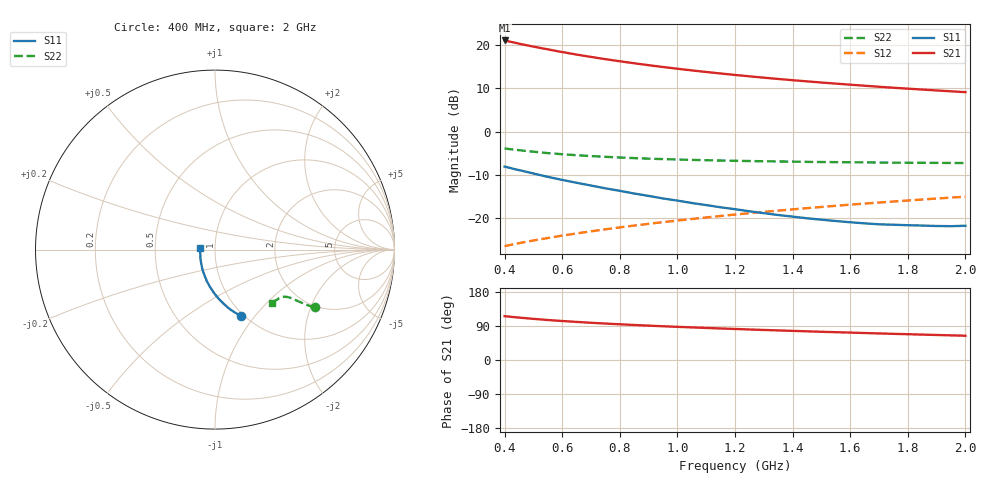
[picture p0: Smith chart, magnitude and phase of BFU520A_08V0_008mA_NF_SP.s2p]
! Filename:  P:\Prog\Test\Noise\ATS_data\Testdata_Net\06 Compressed Noise after Statistics\BFU520A_APG2013_30_A05_08p0V_008mA_NF_CM01_D.sf
! Date/Time: Wed 24/Apr/2013 20:06:19
! BFU520A_APG2013_30_A05_08p0V_1to20mA_NF_CM01_Bias5_R.sf
! Noise Parameter Data File
! BFU520A_APG2013_30_A05_08p0V_1to20mA_NF_CM01
! Date/time: Thu Apr 11 09:33:54 2013
! VAR V_out= 8.000000
! VAR I_out= 8.005000
! VAR V_in= 0.828700
! VAR I_in= 0.085505
! Device data file deembeded for feedlines and parallel
! Original file: \06 Compressed Noise after Statistics\BFU520A_APG2013_30_A05_08p0V_008mA_NF_CM01_R.sf
! Feed-files: PR017V01_150413_Feed1.s2p, PR017V01_150413_Feed2.s2p
! Parallel-file: PR017V01_150413_Par.s2p
# MHz S MA R 50
!  Freq-MHz  S11-mag  S11-arg  S21-mag  S21-arg  S12-mag  S12-arg  S22-mag  S22-arg
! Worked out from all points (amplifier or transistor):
!   37 points, 400 MHz to 2 GHz, reference 50 ohm
!   highest |S21| = 21.1 dB at 400 MHz (marker M1)
!   |S21| within 3 dB of that: start of sweep to 627.7 MHz
!   unconditionally stable (mu >= 1): 1.423 GHz to end of sweep
!   at 500 MHz: K = 0.76, MSG = 22.4 dB, |S12| = -25.1 dB
!   at 1.1 GHz: K = 0.97, MSG = 16.8 dB, |S12| = -19.8 dB
!   at 2 GHz: K = 1.01, MAG = 11.6 dB, |S12| = -15.0 dB
!   lowest NFmin = 0.76 dB at 420 MHz
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400  0.3961 -68.7  11.34 115.7  0.0478 67.2  0.6417 -30.1
420  0.3819 -70.6  10.95 114.1  0.04942 67.1  0.6294 -30.4
440  0.3676 -72.5  10.6 112.6  0.051 67.1  0.6184 -30.6
460  0.3549 -74.1  10.25 111.2  0.05255 67.2  0.6082 -30.9
480  0.3424 -75.9  9.927 109.9  0.05409 67.1  0.5977 -31.1
500  0.3301 -77.5  9.621 108.6  0.05564 67.2  0.589 -31.2
550  0.3016 -81.5  8.949 105.5  0.05936 67.3  0.5673 -31.5
600  0.2785 -85.1  8.326 102.9  0.06325 67.5  0.551 -31.7
650  0.2579 -88.4  7.792 100.5  0.06706 67.8  0.5367 -32.0
700  0.2396 -91.7  7.318 98.2  0.07093 68.1  0.5246 -32.1
750  0.2226 -94.8  6.893 96.2  0.07481 68.3  0.5139 -32.3
800  0.2081 -98.1  6.519 94.3  0.07873 68.5  0.5049 -32.5
850  0.1938 -101.2  6.181 92.4  0.08264 68.7  0.4968 -32.7
950  0.1699 -107.4  5.596 89.0  0.09052 69.0  0.4838 -33.2
1050  0.1507 -113.5  5.114 86.0  0.0985 69.2  0.4737 -33.7
1150  0.1343 -120.5  4.712 83.2  0.1066 69.3  0.4657 -34.4
1200  0.1277 -123.6  4.534 81.9  0.1107 69.4  0.4623 -34.7
1350  0.1094 -134.3  4.073 78.0  0.123 69.3  0.4545 -36.0
1500  0.09674 -146.4  3.705 74.5  0.1355 69.1  0.4476 -37.4
1650  0.08772 -158.4  3.402 71.2  0.1483 68.7  0.4435 -39.1
1750  0.08453 -167.3  3.226 69.1  0.1567 68.4  0.44 -40.2
2000  0.08221 172.2  2.869 64.0  0.1782 67.5  0.4355 -43.5
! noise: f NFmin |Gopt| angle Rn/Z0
400  0.7999  0.07606  14.82  0.1206
460  0.7771  0.05804  24.83  0.1111
600  0.8833  0.06707  21.02  0.1279
800  0.8284  0.03416  61.77  0.1092
1000  0.8395  0.02823  100.7  0.1054
1200  0.9051  0.02822  118.2  0.103
1400  0.9255  0.04798  165.1  0.098
1600  0.9379  0.0693  177.7  0.0931
1800  0.909  0.1293  -166.5  0.0797
2000  0.8805  0.1365  -150.2  0.0954
